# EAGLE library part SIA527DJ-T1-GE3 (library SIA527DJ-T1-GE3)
MOSFET -12V Vds 8V Vgs SC-70 N&P PAIR Source: Datasheet
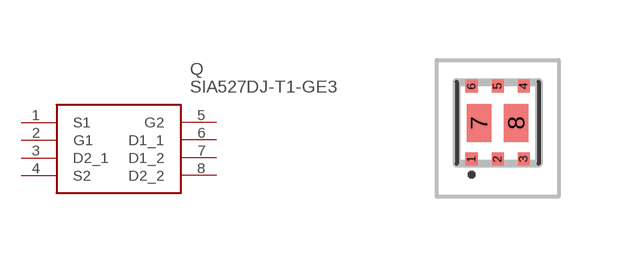
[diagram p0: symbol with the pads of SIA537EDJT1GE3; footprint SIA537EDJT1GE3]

Designator prefix Q

## SIA527DJ-T1-GE3 (Arrow_Part_Number: SIA527DJ-T1-GE3; Arrow_Price-Stock: https://www.arrow.com/en/products/sia527dj-t1-ge3/vishay?region=nac; Description: MOSFET -12V Vds 8V Vgs SC-70 N&P PAIR; Height: 0mm; Manufacturer_Name: Vishay; Manufacturer_Part_Number: SIA527DJ-T1-GE3; Mouser_Part_Number: 78-SIA527DJ-T1-GE3; Mouser_Price-Stock: https://www.mouser.co.uk/ProductDetail/Vishay-Semiconductors/SIA527DJ-T1-GE3?qs=IcBct1gTIwz%2FpGFBQNHwbQ%3D%3D)  [SIA537EDJT1GE3]
1  S1
2  G1
3  D2_1
4  S2
5  G2
6  D1_1
7  D1_2
8  D2_2

## Footprint SIA537EDJT1GE3 (pad centres in mm)
PowerPAK SC-70-6L Dual
smd 0.3 x 0.325: 1 -0.65,-0.912; 2 0,-0.912; 3 0.65,-0.912; 4 0.65,0.913; 5 0,0.913; 6 -0.65,0.913
smd 0.613 x 0.95: 7 -0.466,0; 8 0.466,0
